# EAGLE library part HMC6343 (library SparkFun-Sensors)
Honewell HMC6343 Compass w/ Tilt Compensation The Honeywell HMC6343 is a fully integrated compass module that includes firmware for heading computation and calibration for magnetic distortions. The module combines three-axis magneto-resistive sensor, three-axis MEMS accelerometer, analog and digital support circuits, microprocessor and algorithms required for heading computation Datasheet SparkFun Products SparkFun HMC6343 Breakout (SEN-12916)
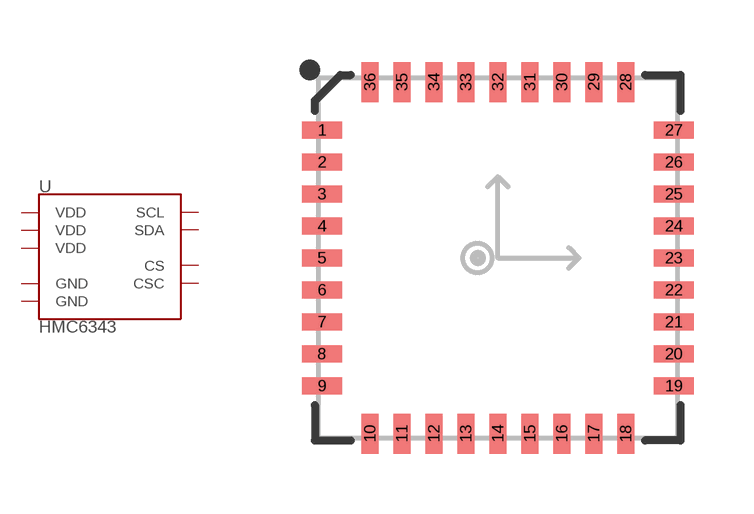
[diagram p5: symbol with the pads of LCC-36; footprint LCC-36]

Designator prefix U

## HMC6343 (PROD_ID: IC-12117)  [LCC-36]
3  VDD
11  VDD
21  VDD
22  CS
25  GND
29  GND
32  SCL
35  CSC
36  SDA

## Footprint LCC-36 (pad centres in mm)
36-Pin LCC (9 x 9 mm) Datasheet Specifications: Pin Count: 36 Area: 9.0 x 9.0 x 1.87 mm Pitch: 0.8 mm Devices Using: HMC6343
smd 1 x 0.42: 1 -4.4,3.2; 2 -4.4,2.4; 3 -4.4,1.6; 4 -4.4,0.8; 5 -4.4,0; 6 -4.4,-0.8; 7 -4.4,-1.6; 8 -4.4,-2.4; 9 -4.4,-3.2; 19 4.4,-3.2; 20 4.4,-2.4; 21 4.4,-1.6; 22 4.4,-0.8; 23 4.4,0; 24 4.4,0.8; 25 4.4,1.6; 26 4.4,2.4; 27 4.4,3.2
smd 0.42 x 1: 10 -3.2,-4.4; 11 -2.4,-4.4; 12 -1.6,-4.4; 13 -0.8,-4.4; 14 0,-4.4; 15 0.8,-4.4; 16 1.6,-4.4; 17 2.4,-4.4; 18 3.2,-4.4; 28 3.2,4.4; 29 2.4,4.4; 30 1.6,4.4; 31 0.8,4.4; 32 0,4.4; 33 -0.8,4.4; 34 -1.6,4.4; 35 -2.4,4.4; 36 -3.2,4.4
